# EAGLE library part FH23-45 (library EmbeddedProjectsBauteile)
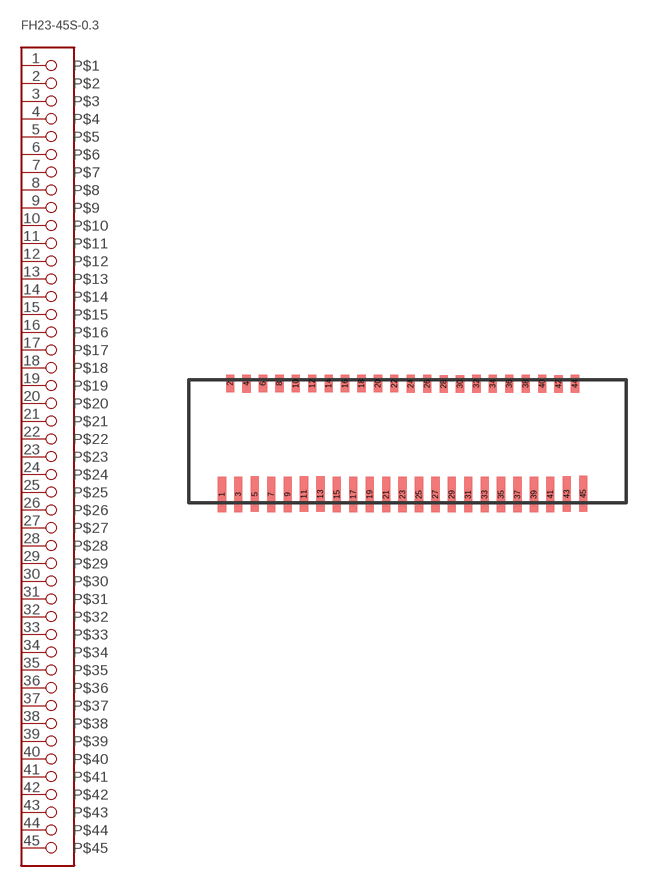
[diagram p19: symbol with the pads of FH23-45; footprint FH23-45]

Designator prefix -

## FH23-45  [FH23-45]
1  P$1
2  P$2
3  P$3
4  P$4
5  P$5
6  P$6
7  P$7
8  P$8
9  P$9
10  P$10
11  P$11
12  P$12
13  P$13
14  P$14
15  P$15
16  P$16
17  P$17
18  P$18
19  P$19
20  P$20
21  P$21
22  P$22
23  P$23
24  P$24
25  P$25
26  P$26
27  P$27
28  P$28
29  P$29
30  P$30
31  P$31
32  P$32
33  P$33
34  P$34
35  P$35
36  P$36
37  P$37
38  P$38
39  P$39
40  P$40
41  P$41
42  P$42
43  P$43
44  P$44
45  P$45

## Footprint FH23-45 (pad centres in mm)
smd 0.3 x 1.3: 1 -6.78,-1.94; 3 -6.18,-1.94; 5 -5.58,-1.93; 7 -4.98,-1.94; 9 -4.38,-1.94; 11 -3.78,-1.93; 13 -3.18,-1.93; 15 -2.58,-1.94; 17 -1.98,-1.94; 19 -1.38,-1.94; 21 -0.78,-1.95; 23 -0.18,-1.95; 25 0.42,-1.95; 27 1.02,-1.94; 29 1.62,-1.95; 31 2.22,-1.95; 33 2.82,-1.95; 35 3.42,-1.95; 37 4.02,-1.95; 39 4.62,-1.95; 41 5.22,-1.94; 43 5.82,-1.93; 45 6.42,-1.92
smd 0.3 x 0.65: 2 -6.48,2.11; 4 -5.88,2.1; 6 -5.28,2.11; 8 -4.68,2.11; 10 -4.08,2.11; 12 -3.48,2.11; 14 -2.88,2.11; 16 -2.28,2.11; 18 -1.68,2.11; 20 -1.08,2.11; 22 -0.48,2.11; 24 0.12,2.1; 26 0.72,2.1; 28 1.32,2.09; 30 1.92,2.09; 32 2.52,2.1; 34 3.12,2.1; 36 3.72,2.1; 38 4.32,2.1; 40 4.92,2.1; 42 5.52,2.09; 44 6.12,2.1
